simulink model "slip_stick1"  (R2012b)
settings: Solver=ode1  StartTime=0.0  StopTime=100  FixedStep=0.001  MaxStep=0.001  RelTol=1e-3
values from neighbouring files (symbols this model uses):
  c = 2200    [coulomb_1.m]    (also in coulomb_10.m = 0.1; coulomb_11.m = 0; coulomb_2.m; coulomb_3.m)
  FG = 500    [coulomb_1.m]    (also in coulomb_10.m = 10; coulomb_11.m = 10; coulomb_2.m; coulomb_3.m)
  FH = 12    [coulomb_10.m]    (also in coulomb_11.m; coulomb_3.m = 600; coulomb_4.m = 600; position_reg_1.m = 3.956)
  k = 10    [coulomb_10.m]    (also in coulomb_11.m; diff_filter_1.m = 250; diff_filter_2.m = 250; dry_friction_1.m = 2200)
  m = 400    [coulomb_1.m]    (also in coulomb_10.m = 10; coulomb_11.m = 10; coulomb_2.m; coulomb_3.m)
  vstr = 0.1    [coulomb_10.m]    (also in coulomb_11.m; coulomb_3.m = 0.05; coulomb_4.m = 0.01; slip_stick_1.m = 0.01)
  vz = -ampl*2*pi*fanr*sin(2*pi*fanr*t)    [foerder_haft_gleit_1.m]    (also in foerder_haft_gleit_2.m; slip_stick_1.m = 0.1; slip_stick_2.m = 0.1; slip_stick_21.m = 0.1)
undefined symbols (not defined in the file or in its folder): sgn

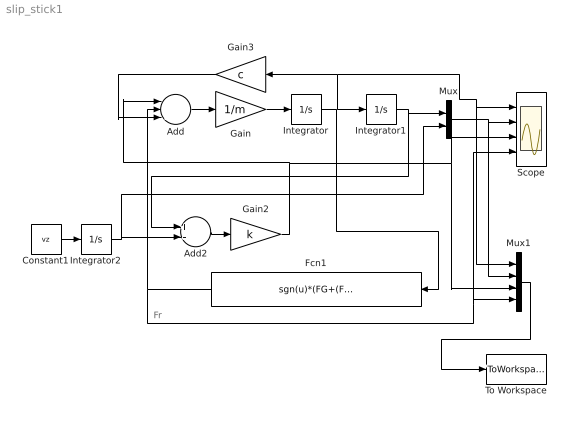
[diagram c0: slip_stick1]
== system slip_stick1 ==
  note: Fr
  Add : Sum  Inputs=---
  Add2 : Sum  Inputs=+-
  Constant1 : Constant  Value=vz
  Fcn1 : Fcn  Expr=sgn(u)*(FG+(FH-FG)*exp(-abs(u/vstr)))
  Gain : Gain  Gain=1/m
  Gain2 : Gain  Gain=k
  Gain3 : Gain  Gain=c
  Integrator : Integrator
  Integrator1 : Integrator
  Integrator2 : Integrator
  Mux : Mux  Inputs=2
  Mux1 : Mux
  Scope : Scope  NumInputPorts=4
  To Workspace : ToWorkspace  VariableName=y  SampleTime=-1  SaveFormat=Structure With Time
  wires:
  Add/1 -> Gain/1
  Gain/1 -> Integrator/1
  Gain3/1 -> Add/3
  Gain2/1 -> Mux1/3, Scope/3, Add/1
  Constant1/1 -> Integrator2/1
  Integrator2/1 -> Mux/2, Add2/2
  Add2/1 -> Gain2/1
  Integrator1/1 -> Mux/1, Add2/1
  Integrator/1 -> Integrator1/1, Mux1/1, Scope/1, Gain3/1, Fcn1/1
  Mux/1 -> Mux1/2, Scope/2
  Fcn1/1 -> Mux1/4, Scope/4, Add/2
  Mux1/1 -> To Workspace/1
